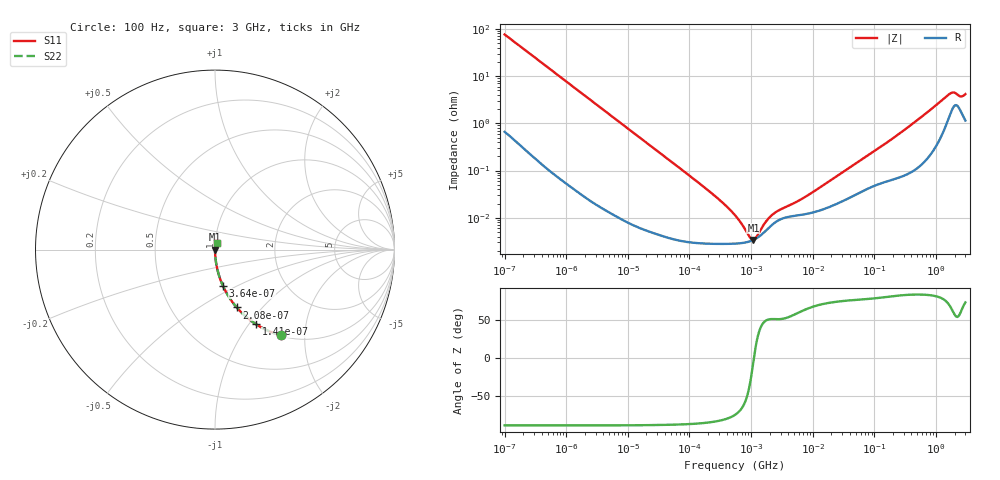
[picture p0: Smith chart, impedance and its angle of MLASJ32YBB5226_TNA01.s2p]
! MLASJ32YBB5226_TNA01  S-PARAMETER MODEL  ( Standard Model )
! Model Generated by TAIYO YUDEN Corporation (http://www.ty-top.com)
! Version 1.0
! TAIYO YUDEN Control No. 220601
! Copyright(c) 2009 TAIYO YUDEN CO.,LTD. All Rights Reserved.
! Product Description (link to TY-COMPAS)
! https://ds.yuden.co.jp/TYCOMPAS/or/detail?pn=MLASJ32YBB5226MTNA01&u=M
! Products Name : Multilayer Ceramic Capacitors
! Characteristics :
!  Capacitance : 22 [uF] , Rated Voltage : 6.3 [V] , TCC : B / X5R
!  Case Size : 3.2 x 2.5 / 0.126 x 0.098 [mm/inch] , Thickness : 1.9 / 0.075 [mm/inch]
!  (Conditions: Temperature = 25 [degC] , DC Bias Voltage = 0 [V])
! External Node Assignments :
!  1  o---| |---o  2
! GND o---------o GND
! Frequency Range : 100Hz  -  3GHz  [ 401 STEP ]
# MHZ S RI R 50
! Freq[MHz].  S11 Real  S11 Imag  S21 Real  S21 Imag  S12 Real  S12 Imag  S22 Real  S22 Imag
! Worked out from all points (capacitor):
!   401 points, 100 Hz to 3 GHz, reference 50 ohm
!   read as one part in series: C = 20.9 uF near 109 Hz
!   lowest |Z| = 3.39 mohm at 1.091 MHz (marker M1)
!   series resonance near 1.11 MHz, so ESL is about 980 pH
!   S11 on the Smith chart (normalised r, x): 100 Hz: 1.01, -1.52; 141 Hz: 1.01, -1.08; 208 Hz: 1.01, -0.74; 364 Hz: 1.00, -0.42; 3 GHz: 1.02, +0.08
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0.0001  0.3678 -0.4779  0.6322 0.4779  0.6322 0.4779  0.3678 -0.4779
0.000141  0.228 -0.4154  0.772 0.4154  0.772 0.4154  0.228 -0.4154
0.000208  0.121 -0.3222  0.879 0.3222  0.879 0.3222  0.121 -0.3222
0.000364  0.0438 -0.2011  0.9562 0.2011  0.9562 0.2011  0.0438 -0.2011
0.000756  0.0109 -0.1004  0.9891 0.1004  0.9891 0.1004  0.0109 -0.1004
0.001788  0.00216 -0.043  0.9978 0.043  0.9978 0.043  0.00216 -0.043
0.031977  4.91e-05 -0.00244  1 0.00244  1 0.00244  4.91e-05 -0.00244
0.231582  2.81e-05 -0.000325  1 0.000325  1 0.000325  2.81e-05 -0.000325
0.388167  2.79e-05 -0.000179  1 0.000179  1 0.000179  2.79e-05 -0.000179
0.547723  2.83e-05 -0.00011  1 0.00011  1 0.00011  2.83e-05 -0.00011
0.650627  2.88e-05 -8.05e-05  1 8.05e-05  1 8.05e-05  2.88e-05 -8.05e-05
1.09055  3.38e-05 -2.53e-06  1 2.53e-06  1 2.53e-06  3.38e-05 -2.53e-06
1.908323  6e-05 7.5e-05  0.9999 -7.5e-05  0.9999 -7.5e-05  6e-05 7.5e-05
2.81117  8.89e-05 0.000113  0.9999 -0.000113  0.9999 -0.000113  8.89e-05 0.000113
5.597215  0.000112 0.000191  0.9999 -0.000191  0.9999 -0.000191  0.000112 0.000191
9.794414  0.000128 0.000317  0.9999 -0.000317  0.9999 -0.000317  0.000128 0.000317
175.1444  0.000627 0.0042  0.9994 -0.0042  0.9994 -0.0042  0.000627 0.0042
513.708  0.0013 0.012  0.9987 -0.012  0.9987 -0.012  0.0013 0.012
1642.185  0.0151 0.0381  0.9849 -0.0381  0.9849 -0.0381  0.0151 0.0381
1950.712  0.0236 0.037  0.9764 -0.037  0.9764 -0.037  0.0236 0.037
2525.516  0.0185 0.0313  0.9815 -0.0313  0.9815 -0.0313  0.0185 0.0313
3000  0.0128 0.039  0.9872 -0.039  0.9872 -0.039  0.0128 0.039
